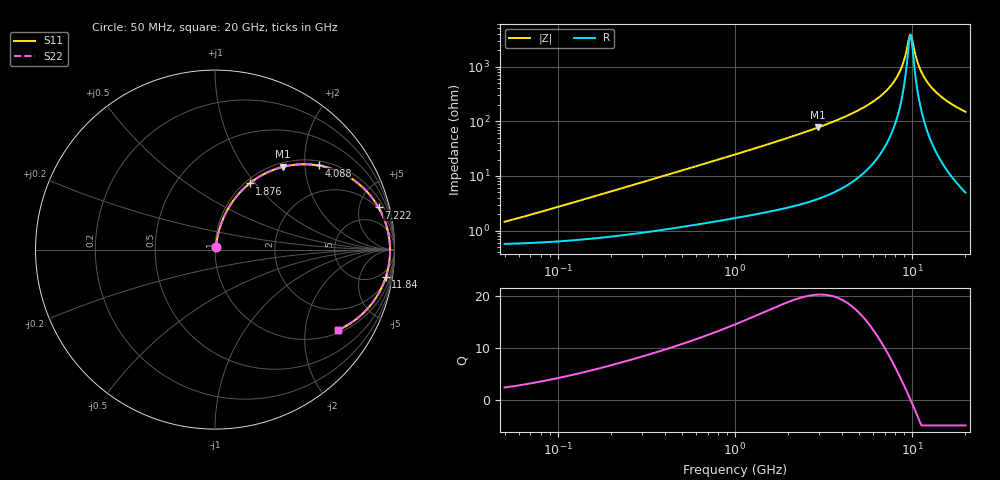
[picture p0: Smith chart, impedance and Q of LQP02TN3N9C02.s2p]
!Murata Part Number: LQP02TN3N9C02
!These Parameters are Measured in Series Mode Connection
!  o--[Z]--o
!Port1  Port2
!  o-------o
!Freq. Start=50[MHz] Stop=20[GHz], 401[Steps]
# Hz S RI R 50
!Freq.(Hz) S11(Real) S11(Imag) S21(Real) S21(Imag) S12(Real) S12(Imag) S22(Real) S22(Imag)
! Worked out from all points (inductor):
!   401 points, 50 MHz to 20 GHz, reference 50 ohm
!   read as one part in series: L = 4.22 nH near 66.46 MHz
!   highest Q = 20.3 at 2.94 GHz (marker M1), where L = 4.17 nH
!   self-resonance near 9.745 GHz
!   S11 on the Smith chart (normalised r, x): 50 MHz: 1.01, +0.03; 1.876 GHz: 1.05, +0.94; 4.088 GHz: 1.12, +2.35; 7.222 GHz: 1.81, +7.44; 11.84 GHz: 3, -12; 20 GHz: 1.10, -2.99
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5e7  0.00586 0.0132  0.9941 -0.0132  0.9941 -0.0132  0.00586 0.0132
1.364002e8  0.00807 0.0352  0.9919 -0.0352  0.9919 -0.0352  0.00807 0.0352
3.721004e8  0.0185 0.0915  0.9815 -0.0915  0.9815 -0.0915  0.0185 0.0915
1e9  0.0714 0.2253  0.9286 -0.2253  0.9286 -0.2253  0.0714 0.2253
1.875929e9  0.1927 0.3684  0.8073 -0.3684  0.8073 -0.3684  0.1927 0.3684
2.728004e9  0.3406 0.4498  0.6594 -0.4498  0.6594 -0.4498  0.3406 0.4498
2.940159e9  0.3789 0.4611  0.6211 -0.4611  0.6211 -0.4611  0.3789 0.4611
4.087748e9  0.5772 0.4686  0.4228 -0.4686  0.4228 -0.4686  0.5772 0.4686
5.683258e9  0.7897 0.3749  0.2103 -0.3749  0.2103 -0.3749  0.7897 0.3749
7.222371e9  0.9112 0.2352  0.0888 -0.2352  0.0888 -0.2352  0.9112 0.2352
7.442007e9  0.9226 0.2141  0.0774 -0.2141  0.0774 -0.2141  0.9226 0.2141
8.141811e9  0.9506 0.1475  0.0494 -0.1475  0.0494 -0.1475  0.9506 0.1475
8.644534e9  0.9636 0.1006  0.0364 -0.1006  0.0364 -0.1006  0.9636 0.1006
9.041845e9  0.9702 0.0646  0.0298 -0.0646  0.0298 -0.0646  0.9702 0.0646
9.600142e9  0.9748 0.0159  0.0252 -0.0159  0.0252 -0.0159  0.9748 0.0159
9.745021e9  0.9751 0.00368  0.0249 -0.00368  0.0249 -0.00368  0.9751 0.00368
1.004137e10  0.9749 -0.0208  0.0251 0.0208  0.0251 0.0208  0.9749 -0.0208
1.098561e10  0.9669 -0.0939  0.0331 0.0939  0.0331 0.0939  0.9669 -0.0939
1.183995e10  0.9518 -0.1531  0.0482 0.1531  0.0482 0.1531  0.9518 -0.1531
1.295331e10  0.9243 -0.2205  0.0757 0.2205  0.0757 0.2205  0.9243 -0.2205
1.460232e10  0.8731 -0.3017  0.1269 0.3017  0.1269 0.3017  0.8731 -0.3017
2e10  0.685 -0.4481  0.315 0.4481  0.315 0.4481  0.685 -0.4481
